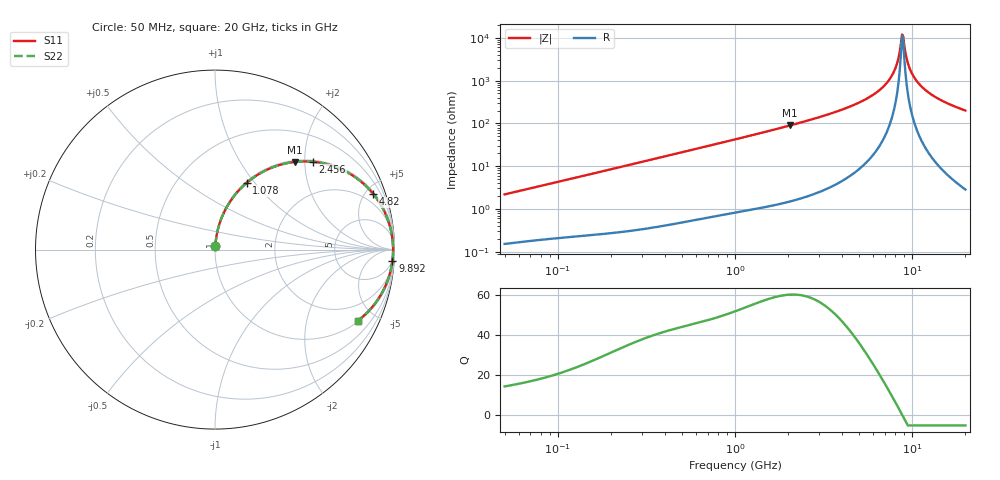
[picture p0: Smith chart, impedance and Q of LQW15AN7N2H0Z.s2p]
!Murata Part Number: LQW15AN7N2H0Z
!These Parameters are Measured in Series Mode Connection
!  o--[Z]--o
!Port1  Port2
!  o-------o
!Freq. Start=50[MHz] Stop=20[GHz], 401[Steps]
# Hz S RI R 50
!Freq.(Hz) S11(Real) S11(Imag) S21(Real) S21(Imag) S12(Real) S12(Imag) S22(Real) S22(Imag)
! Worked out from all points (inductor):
!   401 points, 50 MHz to 20 GHz, reference 50 ohm
!   read as one part in series: L = 6.89 nH near 51.52 MHz
!   highest Q = 60 at 2.052 GHz (marker M1), where L = 6.96 nH
!   self-resonance near 8.775 GHz
!   S11 on the Smith chart (normalised r, x): 50 MHz: 1.00, +0.04; 1.078 GHz: 1.02, +0.91; 2.456 GHz: 1.04, +2.20; 4.82 GHz: 1.15, +5.67; 9.892 GHz: 5, -31; 20 GHz: 1.06, -3.99
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5e7  0.00199 0.0217  0.998 -0.0217  0.998 -0.0217  0.00199 0.0217
1.364002e8  0.00566 0.0576  0.9943 -0.0576  0.9943 -0.0576  0.00566 0.0576
3.721004e8  0.0276 0.1519  0.9724 -0.1519  0.9724 -0.1519  0.0276 0.1519
1e9  0.1556 0.3529  0.8444 -0.3529  0.8444 -0.3529  0.1556 0.3529
1.077769e9  0.176 0.3715  0.824 -0.3715  0.824 -0.3715  0.176 0.3715
2.05233e9  0.4471 0.4889  0.5529 -0.4889  0.5529 -0.4889  0.4471 0.4889
2.456456e9  0.5471 0.4894  0.4529 -0.4894  0.4529 -0.4894  0.5471 0.4894
2.728004e9  0.6066 0.48  0.3934 -0.48  0.3934 -0.48  0.6066 0.48
4.81993e9  0.883 0.3085  0.117 -0.3085  0.117 -0.3085  0.883 0.3085
6.217679e9  0.9555 0.186  0.0445 -0.186  0.0445 -0.186  0.9555 0.186
7.442007e9  0.9835 0.0918  0.0165 -0.0918  0.0165 -0.0918  0.9835 0.0918
8.141811e9  0.9903 0.0436  0.00966 -0.0436  0.00966 -0.0436  0.9903 0.0436
8.644534e9  0.9922 0.0113  0.00777 -0.0113  0.00777 -0.0113  0.9922 0.0113
8.774992e9  0.9924 0.00318  0.00764 -0.00318  0.00764 -0.00318  0.9924 0.00318
8.907419e9  0.9924 -0.00492  0.00763 0.00492  0.00763 0.00492  0.9924 -0.00492
9.041845e9  0.9922 -0.013  0.00776 0.013  0.00776 0.013  0.9922 -0.013
9.457416e9  0.9911 -0.0373  0.00894 0.0373  0.00894 0.0373  0.9911 -0.0373
9.892087e9  0.9887 -0.0615  0.0113 0.0615  0.0113 0.0615  0.9887 -0.0615
1.098561e10  0.9785 -0.1176  0.0215 0.1176  0.0215 0.1176  0.9785 -0.1176
1.257102e10  0.9557 -0.1881  0.0443 0.1881  0.0443 0.1881  0.9557 -0.1881
1.550395e10  0.8987 -0.2908  0.1013 0.2908  0.1013 0.2908  0.8987 -0.2908
2e10  0.796 -0.3959  0.204 0.3959  0.204 0.3959  0.796 -0.3959
